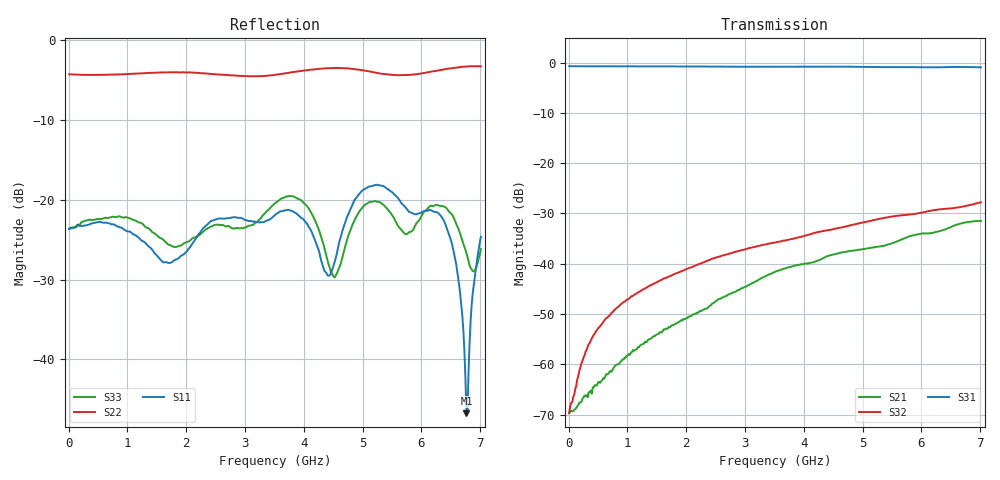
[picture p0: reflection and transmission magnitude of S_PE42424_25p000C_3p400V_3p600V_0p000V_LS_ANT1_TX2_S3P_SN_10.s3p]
! Device ID: PE42424
! Device ID: PE42424
! File Path: z:\PE42424\Characterization\RAW\25p000C\3p400\LS_ANT1_TX2\PE42424_25p000C_3p400V_3p600V_0p000V_LS_ANT1_TX2_S3P_SN_10_.s3p
! Serial: 10
! Lot:
! Temp: 25.000C
! VDD: 3.400
! VSS: 0.000
! Control_Hi: 3.600
! Control_Lo: 0.000
! Logic State: LS_ANT1_TX2
! Port 1: RFC
! Port 2: RF1
! Port 3: RF2
! ThroughPath:1-3
! IDD: 0.0001268915
! ISS: -1.171e-007
#  Hz  S  RI  R  50
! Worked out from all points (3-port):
!   401 points, 10 MHz to 7.01 GHz, reference 50 ohm
!   strongest paths, dB at 10 MHz, 1.76 GHz, 3.51 GHz, 5.26 GHz, 7.01 GHz:
!     S31: -0.7, -0.8, -0.8, -0.9, -0.9
!     S32: -69.7, -42.3, -35.8, -31.1, -27.8
!     S21: -69.6, -52.2, -41.6, -36.6, -31.5
!   lowest |S11| = -46.7 dB at 6.765 GHz (marker M1), VSWR 1.01, Z = 50.3 - j0.376 ohm
!   |S11| at or under -10 dB: start of sweep to end of sweep
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1e7  0.0659 -0.000568  0.000318 5.55e-06  0.9202 -0.00331
     0.00033 -6.49e-06  -0.6099 0.00241  0.000319 0.000105
     0.9198 -0.00356  0.000301 0.000123  0.0655 -0.000614
3.775e8  0.0695 0.0134  -0.000315 -0.000435  0.9144 -0.0588
         -0.00032 -0.000445  -0.5997 0.0694  0.000348 0.00169
         0.9162 -0.059  0.000345 0.00168  0.073 0.0163
9.025e8  0.0641 0.0186  -0.00106 -0.000382  0.9062 -0.1359
         -0.00101 -0.000393  -0.5914 0.1496  0.000492 0.00395
         0.9062 -0.1363  0.000521 0.00397  0.075 0.021
3.51e9  0.0798 0.00643  -0.00706 0.0044  0.7635 -0.4906
        -0.00701 0.00441  -0.3786 0.4721  0.00306 0.016
        0.7637 -0.4921  0.00302 0.0159  0.0935 0.0178
4.525e9  0.00568 -0.0406  -0.00806 0.00944  0.6727 -0.6158
         -0.00811 0.00937  -0.3522 0.5676  0.00487 0.0217
         0.6716 -0.6166  0.00489 0.0217  0.0212 -0.0248
5.085e9  -0.0463 -0.11  -0.00774 0.0119  0.6042 -0.6712
         -0.0077 0.012  -0.325 0.55  0.00689 0.0254
         0.6029 -0.6732  0.00686 0.0254  -0.0381 -0.0874
6.2925e9  0.0812 -0.0114  -0.00785 0.0194  0.4634 -0.769
          -0.00766 0.0195  -0.0427 0.6442  0.0136 0.0319
          0.4618 -0.7701  0.0136 0.0318  0.0917 -0.00834
6.59e9  0.0396 -0.00107  -0.0076 0.023  0.4249 -0.7965
        -0.00748 0.0232  -0.0267 0.6717  0.0149 0.0329
        0.4238 -0.7977  0.0148 0.0328  0.0695 -0.0134
6.765e9  0.00268 -0.00374  -0.00589 0.0251  0.3968 -0.8102
         -0.00584 0.0251  -0.028 0.6815  0.0156 0.0344
         0.3961 -0.8116  0.0155 0.0343  0.0378 -0.0267
7.01e9  -0.0505 -0.0298  -0.00292 0.0265  0.3563 -0.8226
        -0.00273 0.0264  -0.0374 0.683  0.0174 0.0369
        0.3552 -0.8233  0.0173 0.0369  -0.023 -0.0433
